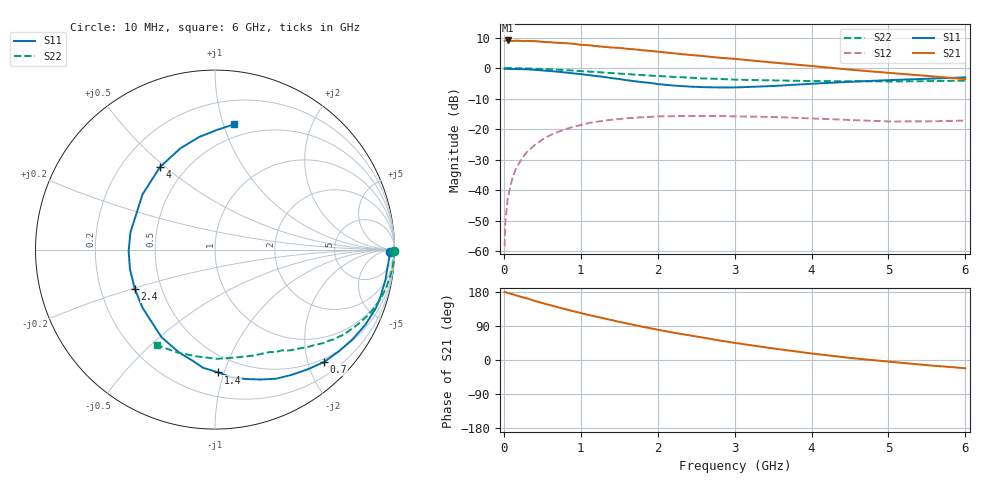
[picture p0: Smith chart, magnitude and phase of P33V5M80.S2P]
! SIEMENS Small Signal Semiconductors
! BFP181
! Si NPN RF Bipolar Junction Transistor in SOT143
! VCE = 3.5 V  IC = 0.8 mA
! Common Emitter S-Parameters:  March  1996
# GHz  S  MA  R  50
!  f  S11  S21  S12  S22
! GHz  MAG  ANG  MAG  ANG  MAG  ANG  MAG  ANG
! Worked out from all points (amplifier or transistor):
!   36 points, 10 MHz to 6 GHz, reference 50 ohm
!   highest |S21| = 9.1 dB at 50 MHz (marker M1)
!   |S21| within 3 dB of that: start of sweep to 1.727 GHz
!   unconditionally stable (mu >= 1): 3.383 GHz to end of sweep
!   at 250 MHz: K = 0.09, MSG = 19.0 dB, |S12| = -29.1 dB
!   at 1.4 GHz: K = 0.46, MSG = 11.8 dB, |S12| = -16.9 dB
!   at 6 GHz: K = 1.32, MAG = 3.4 dB, |S12| = -17.2 dB
!   S11 on the Smith chart (normalised r, x): 10 MHz: 58, -30; 700 MHz: 0.44, -2.30; 1.4 GHz: 0.37, -0.96; 2.4 GHz: 0.35, -0.21; 4 GHz: 0.36, +0.48; 6 GHz: 0.39, +1.08
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0.01  0.973 -0.8  2.8 179.7  0.0012 92.4  0.9991 -0.3
0.02  0.9736 -1.4  2.832 179.4  0.003 86.5  0.9986 -0.6
0.05  0.9711 -3.1  2.838 177.0  0.0073 91.7  0.997 -1.6
0.1  0.9653 -6.6  2.779 174.2  0.0139 84.7  0.9985 -3.1
0.15  0.9649 -9.9  2.814 171.2  0.0213 83.3  0.9948 -4.6
0.25  0.9584 -16.4  2.769 165.2  0.0349 78.8  0.9892 -7.8
0.3  0.9541 -19.8  2.79 162.7  0.0419 76.8  0.9857 -9.3
0.4  0.9372 -26.4  2.776 156.1  0.0544 71.9  0.9772 -12.4
0.7  0.8727 -45.8  2.592 139.4  0.0892 59.6  0.9406 -20.9
0.9  0.8196 -58.2  2.506 128.8  0.1087 51.7  0.9088 -26.0
1.1  0.7674 -70.6  2.372 118.9  0.1248 44.6  0.8769 -30.6
1.4  0.6845 -88.5  2.172 105.4  0.1421 35.0  0.8291 -37.1
1.5  0.6617 -95.8  2.149 100.7  0.1459 32.4  0.8116 -38.8
1.8  0.5881 -114.6  1.966 87.9  0.1561 24.9  0.7674 -43.9
2.2  0.5182 -141.0  1.751 72.2  0.1625 16.0  0.7181 -50.4
2.4  0.4978 -153.8  1.653 65.4  0.1646 12.1  0.6987 -53.5
3  0.4807 168.5  1.417 45.2  0.1614 3.1  0.646 -62.2
3.5  0.5076 142.7  1.233 30.5  0.1578 -2.2  0.6284 -69.9
4  0.5527 123.7  1.081 17.3  0.1492 -5.9  0.6123 -79.0
4.5  0.5961 108.9  0.942 5.5  0.141 -8.0  0.6087 -89.1
5.5  0.6675 88.9  0.744 -13.6  0.1334 -3.8  0.6102 -110.2
6  0.7051 81.5  0.659 -21.8  0.1379 -1.9  0.6226 -121.2
